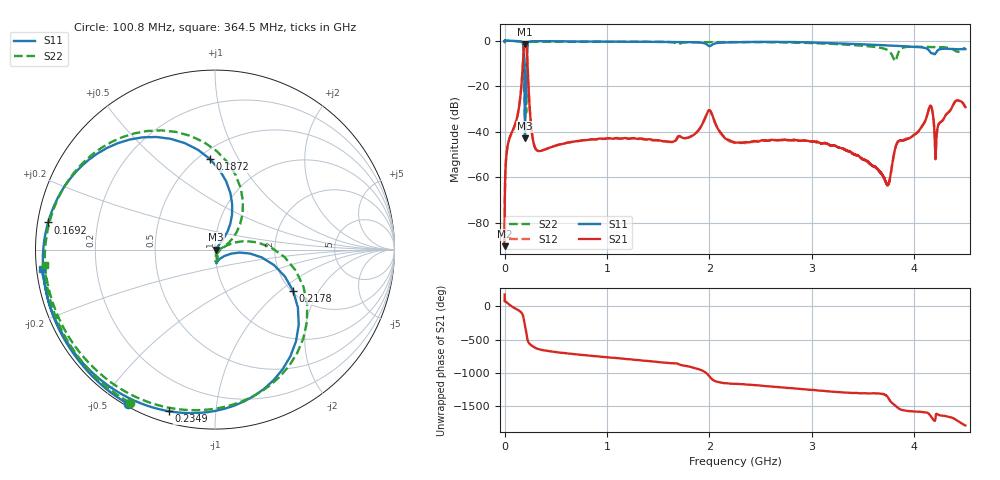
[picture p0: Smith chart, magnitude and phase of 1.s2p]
#  HZ  S  DB  R  50.00
! Rohde & Schwarz Vector Network Analyzer
! Rohde-Schwarz,ZNL6-2Port,1323001206101378,1.50.1.34-21.10.1.104
! Created: UTC 4/19/2023, 7:40:24 AM
! freq[Hz]  db:S11  ang:S11  db:S21  ang:S21  db:S12  ang:S12  db:S22  ang:S22
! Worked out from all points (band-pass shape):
!   5001 points, 5 kHz to 4.5 GHz, reference 50 ohm
!   highest |S21| = -1.42 dB at 199.8 MHz (marker M1); lowest = -90.2 dB at 5 kHz (marker M2)
!   |S21| within 3 dB of the highest: 185.6 MHz to 218.1 MHz (32.45 MHz wide, 16.1 % of centre)
!   lowest |S11| = -42.8 dB at 198.9 MHz (marker M3), VSWR 1.01, Z = 50.7 + j0.05 ohm
!   |S11| at or under -10 dB: 190 MHz to 215.8 MHz (25.71 MHz wide, 12.7 % of centre)
!   |S22| runs from -40.0 to 0.0 dB; largest |S21 - S12| = 0.012
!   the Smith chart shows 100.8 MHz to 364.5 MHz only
!   S11 on the Smith chart (normalised r, x): 100.8 MHz: 0.01, -0.58; 169.2 MHz: 0.03, +0.08; 187.2 MHz: 0.56, +0.77; 217.8 MHz: 2.04, -1.24; 234.9 MHz: 0.05, -0.75; 364.5 MHz: 0.01, -0.06
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5000  0.00 0.0  -90.19 178.9  -88.20 71.8  -0.01 -0.0
3.150496e7  -0.04 -46.6  -45.70 44.9  -45.67 44.0  -0.05 -45.2
1.008049e8  -0.11 -119.4  -37.00 -27.5  -37.05 -29.0  -0.21 -119.2
1.692048e8  -0.52 170.7  -16.72 -104.3  -16.75 -105.4  -0.65 166.3
1.872048e8  -5.90 93.4  -3.45 167.6  -3.46 166.8  -6.18 81.8
1.989048e8  -42.82 3.9  -1.42 71.3  -1.45 70.7  -40.01 -51.3
1.998048e8  -39.71 -52.7  -1.42 64.6  -1.45 64.0  -37.97 -64.6
2.178048e8  -6.15 -27.9  -4.21 -91.0  -4.25 -91.9  -6.66 -14.6
2.349047e8  -0.57 -106.1  -21.89 176.5  -21.94 174.8  -0.82 -101.3
2.826047e8  -0.25 -148.7  -44.83 113.1  -44.88 111.3  -0.46 -147.9
3.645046e8  -0.25 -173.5  -48.24 66.0  -48.22 65.7  -0.43 -174.9
7.506042e8  -0.36 132.3  -43.83 -7.4  -43.78 -6.2  -0.48 125.7
1.500303e9  -0.52 59.1  -43.67 -114.8  -43.90 -117.1  -0.52 48.9
1.998003e9  -2.38 11.9  -30.55 34.0  -30.46 32.3  -0.65 4.9
2.250002e9  -0.67 -9.6  -44.76 -81.3  -44.64 -83.7  -0.57 -19.5
3.000602e9  -0.79 -105.5  -44.29 -173.5  -44.23 -173.5  -1.06 -105.3
3.466801e9  -1.54 -176.1  -50.91 135.5  -50.95 136.6  -2.13 -175.2
3.750301e9  -2.12 142.5  -62.96 58.1  -62.94 58.9  -4.43 105.5
3.805201e9  -2.22 134.5  -49.15 -37.2  -49.32 -35.3  -8.52 16.3
3.845701e9  -2.33 129.1  -44.23 -88.5  -43.87 -89.7  -5.24 -118.6
4.0698e9  -2.91 97.9  -37.93 -143.7  -37.96 -144.1  -2.72 124.4
4.5e9  -3.71 63.9  -29.13 12.5  -29.27 12.7  -3.11 63.9
